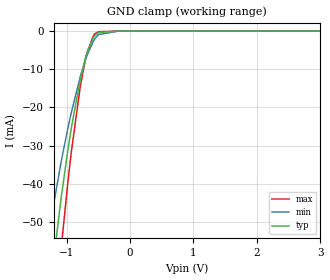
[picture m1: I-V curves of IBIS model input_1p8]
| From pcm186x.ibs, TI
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|   input_1p8 Model
[Model]   input_1p8
Model_type   Input
Vinl = 0.54
Vinh = 1.26
|   typ   min   max
|   (nom PVT)   (fast PVT)   (slow PVT)
C_comp   5.485e-12   5.435e-12   5.485e-12
[Model spec]
|subparameter
Vinl   0.54   0.486   0.594
Vinh   1.26   1.134   1.386
| Where nom  PVT is Nominal Process, 1.8V, 27C
|   Fast PVT is Strong Process,  1.98V, -40C
|   Slow PVT is Weak Process,   1.62V, 125C
[Voltage Range]   1.8   1.62   1.98
|Junction Temperature
[Temperature Range]   27   125   -40
[Power Clamp Reference]   1.8   1.62   1.98
[GND Clamp Reference]   0   0   0
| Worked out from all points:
|   GND clamp passes 1 mA (typ) near -0.54 V on its own axis
[GND Clamp]
|   Voltage   I(typ)   I(min)   I(max)
-1.8V     -273.7mA   -167mA     -385.8mA
-1.291V   -72.63mA   -54.03mA   -97.39mA
-1.244V   -65.49mA   -49.2mA    -87.4mA
-1.079V   -43.03mA   -33.79mA   -56.05mA
-981.9mV  -31.51mA   -25.71mA   -40.07mA
-926.8mV  -25.61mA   -21.5mA    -31.96mA
-778.3mV  -12.3mA    -11.65mA   -14.04mA
-677.3mV  -5.739mA   -6.384mA   -5.692mA
-576.4mV  -1.69mA    -2.616mA   -1.181mA
-497.5mV  -375.4uA   -927.5uA   -162.1uA
-180mV    -17.41nA   -721.8nA   0A
3.6V      0A         0A         0A
[POWER Clamp]
|   Voltage   I(typ)   I(min)   I(max)
-1.8V     0A         0A         0A
0V        0A         0A         0A
3.6V      0A         0A         0A
